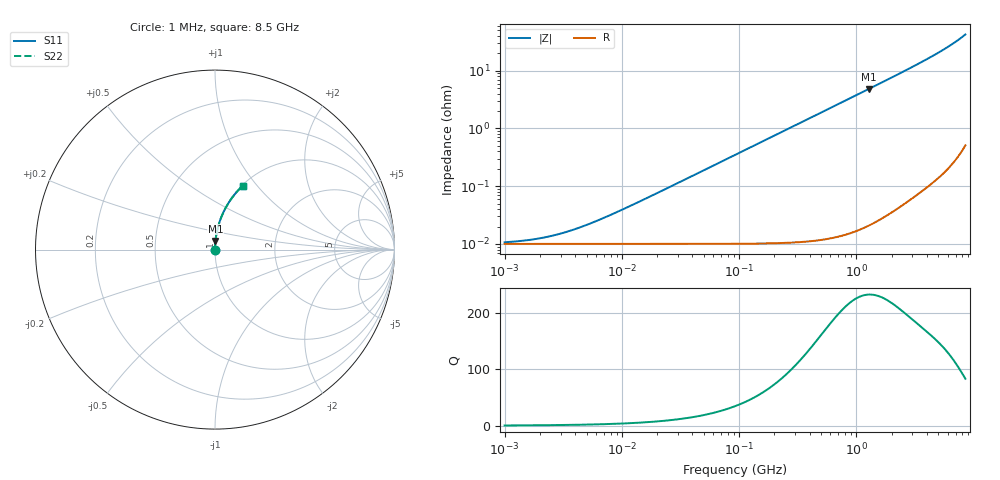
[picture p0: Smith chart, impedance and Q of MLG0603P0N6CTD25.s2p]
! S-Parameter Data Generated by TDK Corporation
! Copyright(C) 2025 TDK Corporation.
! All Rights Reserved.
! TDK P/N: MLG0603P0N6CTD25 (SMD / SMT Inductor (Coil))
! Property: L=0.6nH at 500MHz
! Size(LxWxT): 0.6x0.3x0.3mm
! Model Type: s2p (Touchstone File Format Version 1.0)
! Frequency: DC=Yes Start=1MHz Stop=8500MHz 198points Log-sweep
! Model Generated on Feb. 6, 2025
! Terms and conditions regarding TDK Simulation Models:
! 1)This simulation model is being provided solely for informational
!  purposes. Please refer to the specifications of the products in
!  terms of detailed characteristics of such products.
! 2)In no event shall TDK Corporation of any of its subsidiaries be
!  liable for any loss or damage arising, directly or indirectly,
!  from any information contained in this simulation model, including,
!  but not limited to loss or damages arising from any inaccuracies,
!  omissions or errors in connection with such information.
! 3)Any and all copyrights on this simulation model are owned by
!  TDK Corporation.  Duplication or redistribution of this simulation
!  model without prior written permission from TDK Corporation
!  is prohibited.
! 4)This simulation model is subject to any modification or change
!  without any prior notice.
! 5)Neither TDK Corporation nor any of its subsidiaries shall make any
!  warranty, express or implied, including but not limited to the
!  correctness, implied warranties of merchantability and fitness for
!  a particular purpose with respect to this simulation models.
! 6)The use of this simulation model shall be deemed to have consented
!  to the terms and conditions hereof.
! Port Assignments:
!  1 ---@@@--- 2
! Applicable Conditions:
!  Temperature = 25 degC
!  DC Bias Current = 0 A
!  Small Signal Operation
# Hz S MA R 50
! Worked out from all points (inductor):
!   197 points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, 1 MHz to 8.5 GHz, reference 50 ohm
!   read as one part in series: L = 600 pH near 7.983 MHz
!   highest Q = 233 at 1.281 GHz (marker M1), where L = 603 pH
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1000000  0.0001069 20.6  0.9999 -0.0  0.9999 -0.0  0.0001069 20.6
1515069  0.0001151 29.7  0.9999 -0.0  0.9999 -0.0  0.0001151 29.7
2191881  0.0001297 39.5  0.9999 -0.0  0.9999 -0.0  0.0001297 39.5
2636387  0.0001409 44.8  0.9999 -0.0  0.9999 -0.0  0.0001409 44.8
3171038  0.0001558 50.1  0.9999 -0.0  0.9999 -0.0  0.0001558 50.1
4587603  0.0001997 59.9  0.9999 -0.0  0.9999 -0.0  0.0001997 59.9
6051655  0.0002489 66.3  0.9999 -0.0  0.9999 -0.0  0.0002489 66.3
8360083  0.0003304 72.4  0.9999 -0.0  0.9999 -0.0  0.0003304 72.4
2.10461e7  0.0007991 82.8  0.9999 -0.0  0.9999 -0.0  0.0007991 82.8
9.219544e7  0.003474 88.1  0.9999 -0.2  0.9999 -0.2  0.003474 88.1
4.229561e8  0.01594 88.7  0.9998 -0.9  0.9998 -0.9  0.01594 88.7
7.707615e8  0.02908 88.1  0.9994 -1.7  0.9994 -1.7  0.02908 88.1
1.280704e9  0.04843 87.0  0.9986 -2.8  0.9986 -2.8  0.04843 87.0
1.940355e9  0.07376 85.5  0.9969 -4.2  0.9969 -4.2  0.07376 85.5
2.559585e9  0.09799 84.1  0.9947 -5.6  0.9947 -5.6  0.09799 84.1
3.37643e9  0.1309 82.2  0.9907 -7.5  0.9907 -7.5  0.1309 82.2
4.253027e9  0.1678 80.0  0.9848 -9.7  0.9848 -9.7  0.1678 80.0
5.115526e9  0.2063 77.7  0.9771 -11.9  0.9771 -11.9  0.2063 77.7
5.87536e9  0.2424 75.5  0.9683 -14.0  0.9683 -14.0  0.2424 75.5
6.748056e9  0.287 72.8  0.9555 -16.7  0.9555 -16.7  0.287 72.8
7.750377e9  0.3432 69.3  0.9357 -20.1  0.9357 -20.1  0.3432 69.3
8.5e9  0.3893 66.4  0.9165 -22.9  0.9165 -22.9  0.3893 66.4
